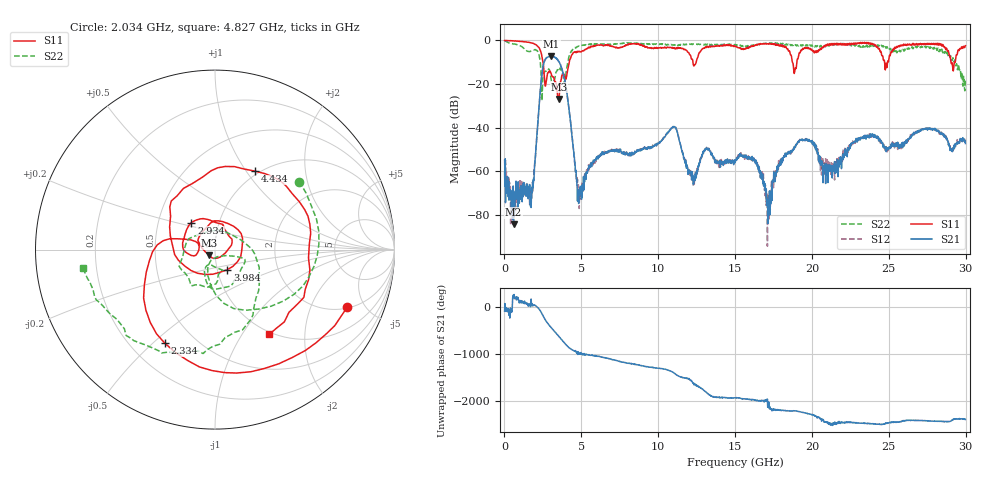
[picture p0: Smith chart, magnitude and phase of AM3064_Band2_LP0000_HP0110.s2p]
# Hz S DB R 50.0
!freq dBS11 angS11 dBS21 angS21 dBS12 angS12 dBS22 angS22
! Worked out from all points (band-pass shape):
!   1600 points, 10 MHz to 29.98 GHz, reference 50 ohm
!   highest |S21| = -7.20 dB at 3.046 GHz (marker M1); lowest = -84.4 dB at 591.1 MHz (marker M2)
!   |S21| within 3 dB of the highest: 2.569 GHz to 3.574 GHz (1.005 GHz wide, 32.7 % of centre)
!   lowest |S11| = -26.8 dB at 3.553 GHz (marker M3), VSWR 1.10, Z = 46.7 - j2.87 ohm
!   |S11| at or under -10 dB: 2.507 GHz to 4.212 GHz (1.705 GHz wide, 50.8 % of centre); 18.73 GHz to 19.02 GHz (290.1 MHz wide, 1.54 % of centre); 29.04 GHz to 29.27 GHz (225.6 MHz wide, 0.774 % of centre)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
!   |S22| runs from -27.6 to -0.2 dB; largest |S21 - S12| = 0.011
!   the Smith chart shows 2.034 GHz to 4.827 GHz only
!   S11 on the Smith chart (normalised r, x): 2.034 GHz: 2.07, -3.73; 2.334 GHz: 0.34, -0.55; 2.934 GHz: 0.74, +0.23; 3.984 GHz: 1.12, -0.25; 4.434 GHz: 0.96, +1.10; 4.827 GHz: 0.97, -1.33
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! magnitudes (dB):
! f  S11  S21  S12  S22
! 10 MHz  0.0  -60.5  -54.6  -0.2
! 591.1 MHz  -0.2  -84.4  -79.8  -1.6
! 1.734 GHz  -1.1  -76.7  -72.4  -4.8
! 2.034 GHz  -1.9  -51.0  -50.7  -4.4
! 2.334 GHz  -4.6  -22.9  -22.8  -10.3
! 2.934 GHz  -14.0  -7.4  -7.4  -13.7
! 3.046 GHz  -15.4  -7.2  -7.2  -18.4
! 3.553 GHz  -26.8  -10.0  -9.8  -12.5
! 3.984 GHz  -17.6  -20.8  -20.7  -16.2
! 4.434 GHz  -6.2  -46.6  -46.6  -4.2
! 4.827 GHz  -5.0  -74.8  -70.9  -2.6
! 5.015 GHz  -5.1  -72.9  -70.3  -2.4
! 10 GHz  -3.4  -47.5  -46.8  -1.7
! 11.09 GHz  -3.9  -39.7  -39.6  -2.0
! 12.32 GHz  -11.8  -63.4  -62.4  -1.6
! 15 GHz  -2.5  -55.9  -55.6  -1.8
! 17.2 GHz  -1.6  -79.3  -78.6  -1.5
! 18.14 GHz  -3.0  -53.8  -53.5  -1.9
! 19.99 GHz  -4.2  -46.8  -46.8  -2.1
! 21.04 GHz  -1.9  -65.2  -58.0  -2.0
! 25 GHz  -9.0  -49.4  -49.3  -3.2
! 29.98 GHz  -2.4  -47.3  -46.7  -17.3
